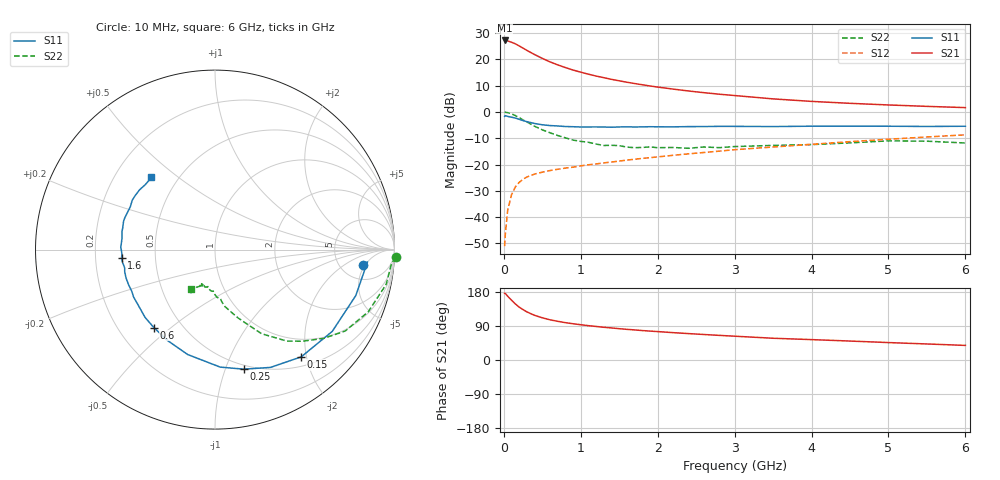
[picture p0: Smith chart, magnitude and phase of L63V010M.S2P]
!  INFINEON TECHNOLOGIES Small Signal Semiconductors
! BFR380L3 , Si-NPN RF-Transistor in TSLP-3-1
!  Vce=3 V,  Ic=10 mA
! Common Emitter S-Parameters:  07. March 2005
#  GHz  S  MA  R  50
! f  S11  S21  S12  S22
! GHz  Mag  Ang  Mag  Ang  Mag  Ang  Mag  Ang
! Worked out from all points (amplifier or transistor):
!   36 points, 10 MHz to 6 GHz, reference 50 ohm
!   highest |S21| = 27.2 dB at 10 MHz (marker M1)
!   |S21| within 3 dB of that: start of sweep to 254.7 MHz
!   unconditionally stable (mu >= 1): 2.154 GHz to 4.75 GHz
!   at 250 MHz: K = 0.26, MSG = 24.9 dB, |S12| = -25.6 dB
!   at 1.4 GHz: K = 0.89, MSG = 15.7 dB, |S12| = -19.0 dB
!   at 6 GHz: K = 0.96, MSG = 5.2 dB, |S12| = -8.7 dB
!   S11 on the Smith chart (normalised r, x): 10 MHz: 8.10, -4.43; 150 MHz: 0.66, -1.91; 250 MHz: 0.46, -1.16; 600 MHz: 0.35, -0.44; 1.6 GHz: 0.31, -0.04; 6 GHz: 0.36, +0.40
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0.01  0.8268 -6.0  22.99 175.8  0.0028 84.9  1.007 -2.4
0.02  0.8525 -4.6  22.77 175.5  0.0049 86.9  0.9856 -4.7
0.05  0.8251 -18.1  22.5 168.3  0.0135 80.7  0.9731 -11.5
0.1  0.7965 -34.9  21.26 157.7  0.0267 74.4  0.9214 -22.1
0.15  0.7668 -51.2  19.82 147.9  0.0376 66.7  0.8558 -32.0
0.2  0.7255 -64.8  18.08 139.5  0.0458 61.6  0.7822 -39.2
0.25  0.6851 -76.5  16.43 132.9  0.0526 56.4  0.7061 -46.3
0.3  0.6552 -87.5  14.86 126.9  0.0581 53.8  0.6474 -51.9
0.4  0.6041 -104.6  12.39 117.8  0.0659 49.4  0.536 -61.0
0.5  0.5716 -117.4  10.49 111.4  0.0717 48.0  0.458 -66.2
0.6  0.552 -128.1  8.992 106.1  0.0769 47.1  0.4025 -71.3
0.8  0.5292 -143.1  7.015 98.5  0.0856 48.0  0.3228 -80.0
0.9  0.5251 -149.6  6.285 95.6  0.0892 48.6  0.2923 -82.7
1.1  0.5198 -158.1  5.24 90.6  0.0991 50.5  0.2655 -87.7
1.4  0.5134 -168.6  4.181 84.6  0.1117 52.8  0.2325 -93.6
1.6  0.5227 -175.1  3.687 80.9  0.1216 54.2  0.2146 -100.4
2.2  0.522 172.9  2.73 72.2  0.15 57.6  0.2113 -105.9
2.8  0.5335 162.7  2.183 65.0  0.1801 59.8  0.2097 -113.6
3.5  0.5287 153.2  1.777 57.4  0.2157 60.0  0.2316 -115.7
4.5  0.5369 146.0  1.463 50.0  0.2728 60.9  0.2585 -118.2
5.5  0.5308 136.9  1.28 42.3  0.3348 59.0  0.2784 -120.2
6  0.5356 131.4  1.213 38.5  0.368 57.4  0.2572 -121.8
